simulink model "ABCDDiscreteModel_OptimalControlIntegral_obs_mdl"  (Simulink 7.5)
settings: Solver=FixedStepDiscrete  StartTime=0.0  StopTime=10.0  FixedStep=Ts  RelTol=1e-3
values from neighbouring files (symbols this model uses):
  H = Ki(n+1)    [TSC140415ProvaMatlab.m]
  K = Ki(1:n)    [TSC140415ProvaMatlab.m]
  L = -acker(A',C',[0 0 0])'    [TSC140415ProvaMatlab.m]
  n = 3    [TSC140415ProvaMatlab.m]
  tp = 2    [TSC140415ProvaMatlab.m]
  Ts = 0.05    [TSC140415ProvaMatlab.m]
  X0 = [0 0 0.5]    [TSC140415ProvaMatlab.m]
  yp = 4    [TSC140415ProvaMatlab.m]
undefined symbols (not defined in the file or in its folder): A, B, C, D, DiscIntNeverNeededParam
libraries: simulink x1

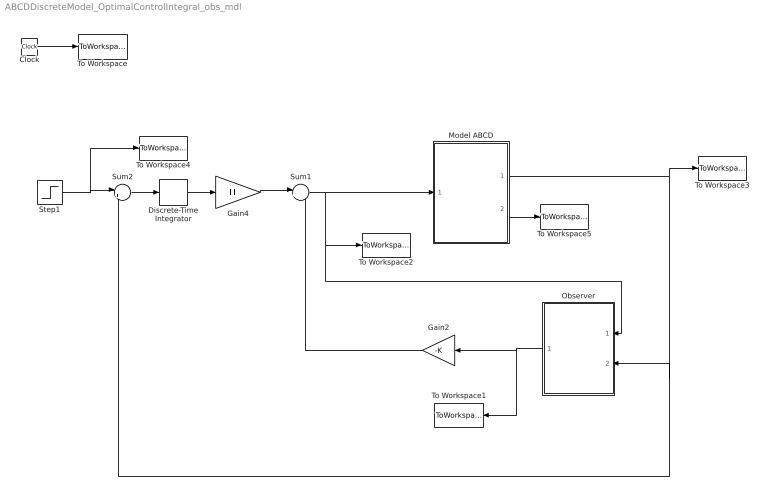
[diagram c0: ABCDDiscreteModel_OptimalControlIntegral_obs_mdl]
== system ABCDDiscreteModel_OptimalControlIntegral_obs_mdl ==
  Clock : Clock
  Discrete-Time Integrator : DiscreteIntegrator  SampleTime=Ts  OutDataType=sfix(16)  OutScaling=2^0  ICPrevOutput=DiscIntNeverNeededParam  ICPrevScaledInput=DiscIntNeverNeededParam
  Gain2 : Gain  Gain=-K  Multiplication=Matrix(K*u)  ParameterDataType=sfix(16)  ParameterScaling=2^0  OutDataType=sfix(16)  OutScaling=2^0
  Gain4 : Gain  Gain=H  Multiplication=Matrix(K*u)  ParameterDataType=sfix(16)  ParameterScaling=2^0  OutDataType=sfix(16)  OutScaling=2^0
  Model ABCD : Subsystem
  Observer : Subsystem
  Step1 : Step  Time=tp  After=yp  SampleTime=0
  Sum1 : Sum  Inputs=|++  OutDataType=sfix(16)  OutScaling=2^0
  Sum2 : Sum  Inputs=|+-  OutDataType=sfix(16)  OutScaling=2^0
  To Workspace : ToWorkspace  VariableName=time  SampleTime=-1  SaveFormat=Array
  To Workspace1 : ToWorkspace  VariableName=Xs  SampleTime=-1  SaveFormat=Array
  To Workspace2 : ToWorkspace  VariableName=u  SampleTime=-1  SaveFormat=Array
  To Workspace3 : ToWorkspace  VariableName=y  SampleTime=-1  SaveFormat=Array
  To Workspace4 : ToWorkspace  VariableName=yd  SampleTime=-1  SaveFormat=Array
  To Workspace5 : ToWorkspace  VariableName=X  SampleTime=-1  SaveFormat=Array
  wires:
  Gain4/1 -> Sum1/1
  Step1/1 -> To Workspace4/1, Sum2/1
  Gain2/1 -> Sum1/2
  Sum1/1 -> Model ABCD/1(U), To Workspace2/1, Observer/1(u)
  Clock/1 -> To Workspace/1
  Model ABCD/1(Y) -> To Workspace3/1, Sum2/2, Observer/2(y)
  Discrete-Time Integrator/1 -> Gain4/1
  Sum2/1 -> Discrete-Time Integrator/1
  Observer/1(Out1) -> Gain2/1, To Workspace1/1
  Model ABCD/2(X) -> To Workspace5/1

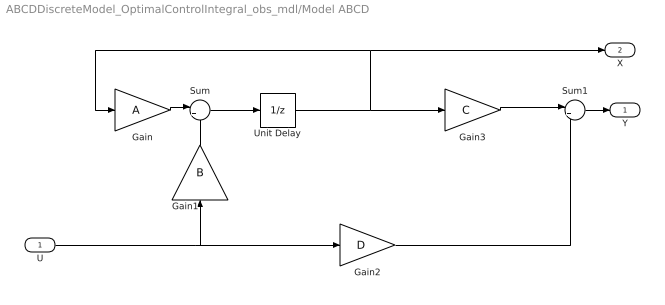
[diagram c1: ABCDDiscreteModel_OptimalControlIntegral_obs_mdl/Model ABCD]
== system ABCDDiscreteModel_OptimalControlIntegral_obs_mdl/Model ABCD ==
  U : Inport
  Gain : Gain  Gain=A  Multiplication=Matrix(K*u)  ParameterDataType=sfix(16)  ParameterScaling=2^0  OutDataType=sfix(16)  OutScaling=2^0
  Gain1 : Gain  Gain=B  Multiplication=Matrix(K*u)  ParameterDataType=sfix(16)  ParameterScaling=2^0  OutDataType=sfix(16)  OutScaling=2^0
  Gain2 : Gain  Gain=D  Multiplication=Matrix(K*u)  ParameterDataType=sfix(16)  ParameterScaling=2^0  OutDataType=sfix(16)  OutScaling=2^0
  Gain3 : Gain  Gain=C  Multiplication=Matrix(K*u)  ParameterDataType=sfix(16)  ParameterScaling=2^0  OutDataType=sfix(16)  OutScaling=2^0
  Sum : Sum  Inputs=|++  OutDataType=sfix(16)  OutScaling=2^0
  Sum1 : Sum  Inputs=|++  OutDataType=sfix(16)  OutScaling=2^0
  Unit Delay : UnitDelay  X0=X0  SampleTime=Ts
  Y : Outport
  X : Outport  Port=2
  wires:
  Gain/1 -> Sum/1
  Gain1/1 -> Sum/2
  Sum/1 -> Unit Delay/1
  Unit Delay/1 -> Gain3/1, Gain/1, X/1
  Gain3/1 -> Sum1/1
  U/1 -> Gain1/1, Gain2/1
  Gain2/1 -> Sum1/2
  Sum1/1 -> Y/1

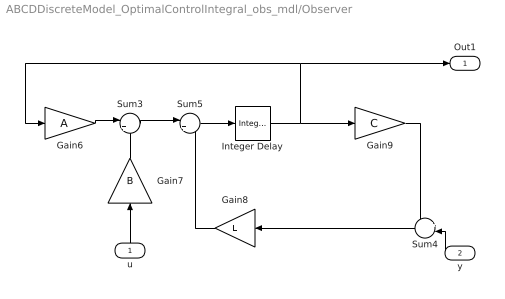
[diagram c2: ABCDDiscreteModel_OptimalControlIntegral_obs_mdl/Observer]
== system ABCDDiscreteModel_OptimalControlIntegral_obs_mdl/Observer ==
  u : Inport
  y : Inport  Port=2
  Gain6 : Gain  Gain=A  Multiplication=Matrix(K*u)  ParameterDataType=sfix(16)  ParameterScaling=2^0  OutDataType=sfix(16)  OutScaling=2^0
  Gain7 : Gain  Gain=B  Multiplication=Matrix(K*u)  ParameterDataType=sfix(16)  ParameterScaling=2^0  OutDataType=sfix(16)  OutScaling=2^0
  Gain8 : Gain  Gain=L  Multiplication=Matrix(K*u)  ParameterDataType=sfix(16)  ParameterScaling=2^0  OutDataType=sfix(16)  OutScaling=2^0
  Gain9 : Gain  Gain=C  Multiplication=Matrix(K*u)  ParameterDataType=sfix(16)  ParameterScaling=2^0  OutDataType=sfix(16)  OutScaling=2^0
  Integer Delay : simulink/Discrete/Integer Delay  vinit=zeros(1,n)  samptime=Ts  NumDelays=1
  Sum3 : Sum  Inputs=|++  OutDataType=sfix(16)  OutScaling=2^0
  Sum4 : Sum  Inputs=+-  OutDataType=sfix(16)  OutScaling=2^0
  Sum5 : Sum  Inputs=|++  OutDataType=sfix(16)  OutScaling=2^0
  Out1 : Outport
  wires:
  Gain6/1 -> Sum3/1
  Integer Delay/1 -> Gain9/1, Gain6/1, Out1/1
  Gain7/1 -> Sum3/2
  Sum4/1 -> Gain8/1
  Gain9/1 -> Sum4/1
  Gain8/1 -> Sum5/2
  Sum3/1 -> Sum5/1
  Sum5/1 -> Integer Delay/1
  u/1 -> Gain7/1
  y/1 -> Sum4/2
